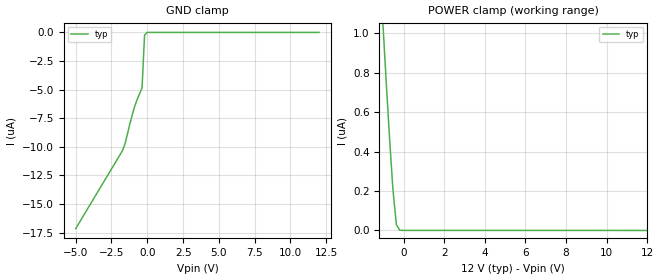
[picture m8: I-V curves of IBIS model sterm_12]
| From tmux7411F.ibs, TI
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| sterm_12
[Model]   sterm_12
Model_type   Terminator
|   typ   min   max
C_comp   4.014581e-12   NA   NA
[Voltage Range]   12   NA   NA
[Temperature Range]   27   NA   NA
[Power Clamp Reference]   12   NA   NA
[GND Clamp Reference]   0   NA   NA
[GND Clamp]
|   Voltage   I(typ)   I(min)   I(max)
-5V       -17.15uA   NA         NA
-1.909V   -10.71uA   NA         NA
-1.737V   -10.34uA   NA         NA
-1.566V   -9.786uA   NA         NA
-1.222V   -8.02uA    NA         NA
-878.8mV  -6.475uA   NA         NA
-707.1mV  -5.859uA   NA         NA
-363.6mV  -4.835uA   NA         NA
-191.9mV  -241nA     NA         NA
-20.2mV   -435.7pA   NA         NA
12V       333.3pA    NA         NA
[POWER Clamp]
|   Voltage   I(typ)   I(min)   I(max)
-5V       8.864uA    NA         NA
-1.05V    1.093uA    NA         NA
-878.8mV  780.5nA    NA         NA
-707.1mV  480.8nA    NA         NA
-535.4mV  210.2nA    NA         NA
-363.6mV  29.28nA    NA         NA
-191.9mV  684.3pA    NA         NA
12V       -249.1pA   NA         NA
